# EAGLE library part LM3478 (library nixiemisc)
Low-Side N-Channel Controller High Efficiency Switching Regulator
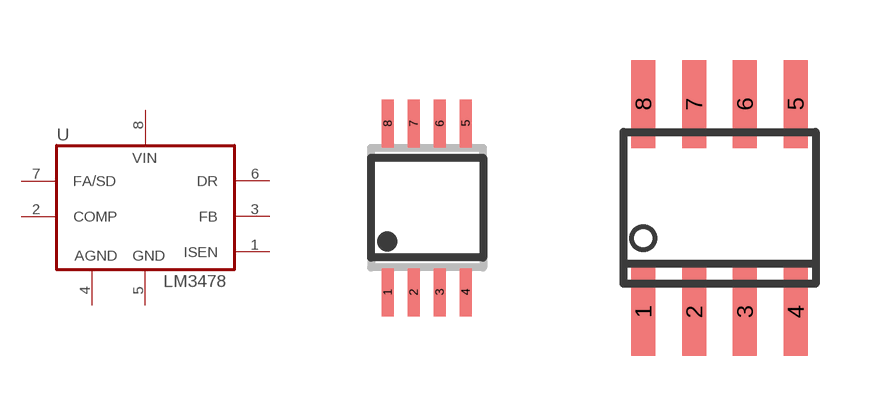
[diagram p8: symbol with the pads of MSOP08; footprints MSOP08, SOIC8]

Designator prefix U

## LM3478  [MSOP08]
1  ISEN  in
2  COMP  in
3  FB  in
4  AGND  pwr
5  PGND  pwr
6  DR  out
7  FA/SD  in
8  VIN  pwr

## LM3478SOIC8  [SOIC8]
Pads as for MSOP08

## Footprint MSOP08 (pad centres in mm)
Mini Small Outline Package
smd 0.3 x 1.2: 1 -0.976,-2.113; 2 -0.326,-2.113; 3 0.324,-2.113; 4 0.974,-2.113; 5 0.974,2.112; 6 0.324,2.112; 7 -0.326,2.112; 8 -0.976,2.112

## Footprint SOIC8 (pad centres in mm)
Small Outline IC
smd 0.6 x 2.2: 1 -1.905,-2.6; 2 -0.635,-2.6; 3 0.635,-2.6; 4 1.905,-2.6; 5 1.905,2.6; 6 0.635,2.6; 7 -0.635,2.6; 8 -1.905,2.6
